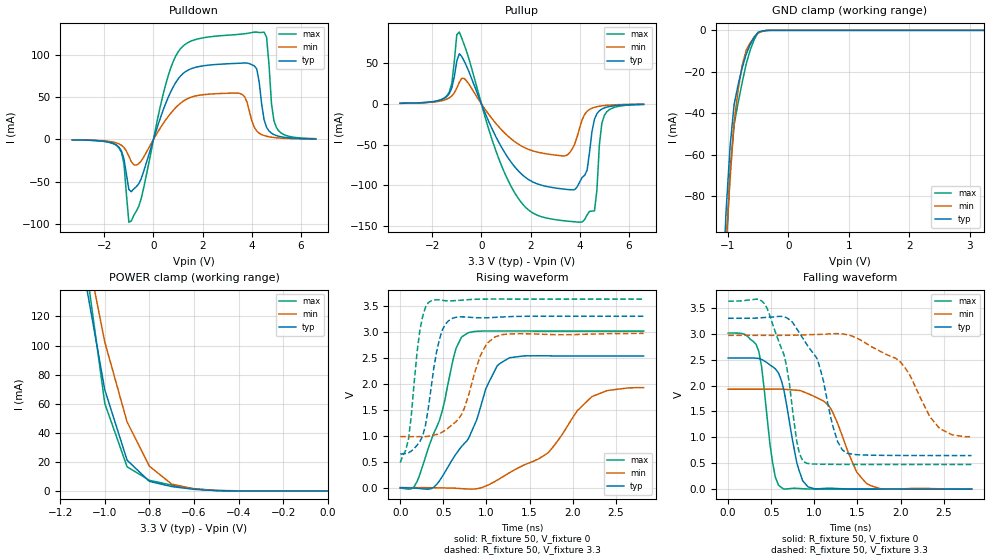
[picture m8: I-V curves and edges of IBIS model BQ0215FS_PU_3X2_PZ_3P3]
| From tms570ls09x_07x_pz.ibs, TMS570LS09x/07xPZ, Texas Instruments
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|   Model Cell BQ0215FS_PU_3X2_PZ_3P3
|BQ0215FS_PU_3X2_PZ_3P3
[Model]   BQ0215FS_PU_3X2_PZ_3P3
Model_type   I/O
Polarity   Non-Inverting
Enable   Active-Low
Vinl =  1.25
Vinh =  1.65
Cref =  15.0001pF
Rref =  101.0000M
Vref =  0V
Vmeas =  1.65
C_comp   1.2p   1.2p   1.2p
[Model Spec]
Vinl   1.25   1.12   1.38
Vinh   1.65   1.45   1.75
[Temperature Range]   25   155   -40
[Voltage Range]   3.3   2.97   3.63
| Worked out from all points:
|   slope of the pulldown table from 0 to 0.495 V, typ, clamps not added: 11.8 ohm
|   slope of the pullup table from 0 to 0.495 V, typ, clamps not added: 14.3 ohm
|   GND clamp passes 1 mA (typ) near -0.50 V on its own axis
|   POWER clamp passes 1 mA (typ) near -0.59 V on its own axis
|   rising waveform, R_fixture 50, V_fixture 0: 20-80 % time 435ps typ, 716ps min, 312ps max; typ from 0 V to 2.53 V
|   rising waveform, R_fixture 50, V_fixture 3.3: 20-80 % time 153ps typ, 240ps min, 117ps max; typ from 0.648 V to 3.3 V
|   falling waveform, R_fixture 50, V_fixture 0: 20-80 % time 168ps typ, 283ps min, 125ps max; typ from 2.53 V to 0 V
|   falling waveform, R_fixture 50, V_fixture 3.3: 20-80 % time 299ps typ, 472ps min, 225ps max; typ from 3.3 V to 0.648 V
[POWER_clamp]
|   voltage   I(typ)   I(min)   I(max)
-3.3V     2.375A     2.63A      3.153A
-1.1V     156mA      180.2mA    173.4mA
-1.067V   127.2mA    154.3mA    135.6mA
-1.033V   98.41mA    128.4mA    97.92mA
-1V       69.61mA    102.5mA    60.2mA
-900mV    21.12mA    47.41mA    16.6mA
-800mV    6.574mA    17mA       7.307mA
-700mV    2.998mA    4.687mA    3.989mA
-600mV    1.086mA    1.404mA    1.425mA
-500mV    187uA      358uA      203.4uA
0V        430.3pA    12.78nA    319.6pA
[Pulldown]
|   voltage   I(typ)   I(min)   I(max)
-3.3V     -560.7uA   -504.5uA   -563.6uA
-1.4V     -9.199mA   -5.273mA   -10.11mA
-1.2V     -22.91mA   -9.491mA   -28.67mA
-1V       -59mA      -19.85mA   -97.49mA
-900mV    -61.64mA   -26.24mA   -96.13mA
1V        71.11mA    40.13mA    102.9mA
3.5V      89.74mA    54.24mA    123.8mA
4.2V      83.16mA    9.923mA    126.4mA
4.6V      14.26mA    3.714mA    120.5mA
4.8V      7.317mA    2.617mA    42.02mA
5V        4.531mA    1.939mA    13.99mA
6.6V      631.1uA    487.2uA    853.6uA
[Pullup]
|   voltage   I(typ)   I(min)   I(max)
-3.3V     614.6uA    591.9uA    551.1uA
-1.4V     9.028mA    5.738mA    10.01mA
-900mV    61.32mA    26.24mA    87.8mA
500mV     -34.85mA   -20.79mA   -49.88mA
1.4V      -78.76mA   -47.33mA   -111.2mA
3.4V      -104.6mA   -63.81mA   -143.4mA
4V        -95.71mA   -29.08mA   -145mA
4.3V      -81.25mA   -9.188mA   -136.1mA
4.6V      -18.8mA    -4.29mA    -131.2mA
4.8V      -8.576mA   -2.945mA   -49.93mA
5V        -5.064mA   -2.148mA   -14.33mA
6.6V      -672.1uA   -541.9uA   -866.9uA
[GND_clamp]
|   voltage   I(typ)   I(min)   I(max)
-3.3V     -1.951A    -1.627A    -3.261A
-1.1V     -130.1mA   -138.8mA   -166.7mA
-1.033V   -87.45mA   -103.2mA   -108mA
-966.7mV  -55.98mA   -71.77mA   -67.59mA
-900mV    -35.7mA    -44.42mA   -45.59mA
-833.3mV  -26.15mA   -28.61mA   -34.91mA
-766.7mV  -18.08mA   -17mA      -25.14mA
-700mV    -11.5mA    -9.608mA   -16.25mA
-633.3mV  -6.833mA   -5.978mA   -9.491mA
-500mV    -870.8uA   -1.241mA   -1.002mA
-300mV    -1.792uA   -15.69uA   -875.3nA
3.233V    409.6pA    4.016uA    238.5pA
[Ramp]
| variable   typ   min   max
dV/dt_f   1.614303/0.3081234n   1.213543/0.5102112n   1.917904/0.2321188n
dV/dt_r   1.540926/0.4431103n   1.176018/0.7396164n   1.826958/0.3142808n
R_load = 50
[Rising Waveform]
R_fixture = 50
V_fixture = 0
V_fixture_min = 0
V_fixture_max = 0
|   time   V(typ)   V(min)   V(max)
0s        -95.09uV   89.18uV    -8.34mV
196ps     -11.58mV   318.5uV    118.9mV
484ps     204.5mV    -5.043mV   1.456V
648ps     651.2mV    -11.61mV   2.686V
776ps     906.4mV    -25.19mV   2.97V
1.124ns   2.344V     143.2mV    3.016V
1.268ns   2.501V     287.6mV    3.015V
1.716ns   2.537V     670.3mV    3.014V
2.224ns   2.534V     1.754V     3.014V
2.824ns   2.533V     1.925V     3.014V
[Rising Waveform]
R_fixture = 50
V_fixture = 3.3
V_fixture_min = 2.97
V_fixture_max = 3.63
|   time   V(typ)   V(min)   V(max)
0s        648.4mV    982.3mV    482.9mV
96ps      671.7mV    981.6mV    939mV
228ps     888.9mV    981.9mV    3.03V
324ps     1.508V     987.9mV    3.559V
452ps     2.834V     1.035V     3.615V
616ps     3.267V     1.228V     3.599V
744ps     3.287V     1.53V      3.613V
952ps     3.268V     2.617V     3.63V
1.104ns   3.279V     2.905V     3.631V
2.824ns   3.3V       2.969V     3.63V
[Falling Waveform]
R_fixture = 50
V_fixture = 0
V_fixture_min = 0
V_fixture_max = 0
|   time   V(typ)   V(min)   V(max)
0s        2.534V     1.93V      3.014V
356ps     2.523V     1.93V      2.658V
516ps     2.364V     1.93V      507.6mV
616ps     2.106V     1.931V     32.1mV
796ps     512.2mV    1.91V      14.87mV
928ps     41.54mV    1.843V     2.875mV
1.192ns   16.87mV    1.549V     61.76uV
1.492ns   1.447mV    327.8mV    31.81uV
1.604ns   596.8uV    110.7mV    13.26uV
2.824ns   92.22uV    1.329mV    -3.494uV
[Falling Waveform]
R_fixture = 50
V_fixture = 3.3
V_fixture_min = 2.97
V_fixture_max = 3.63
|   time   V(typ)   V(min)   V(max)
0s        3.3V       2.97V      3.63V
452ps     3.319V     2.97V      3.491V
648ps     3.329V     2.97V      2.597V
796ps     3.097V     2.974V     924.8mV
884ps     2.868V     2.978V     525.8mV
1.036ns   2.507V     2.987V     482.5mV
1.38ns    692.5mV    2.982V     476.3mV
2ns       649.9mV    2.452V     475.5mV
2.46ns    648.3mV    1.164V     475.6mV
2.824ns   648.1mV    1.012V     475.6mV
